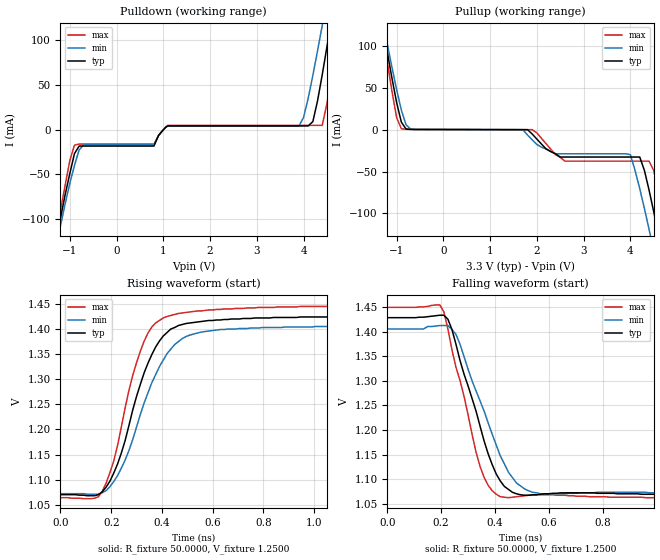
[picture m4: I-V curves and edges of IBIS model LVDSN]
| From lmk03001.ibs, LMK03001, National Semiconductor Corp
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|   Model LVDSN
[Model]  LVDSN
Model_type Output
Polarity   Inverting
Vmeas =  1.2780V
Rref =   50.0000
Vref =   1.2500V
C_comp   1.6000pF   1.6000pF   1.6000pF
[Temperature Range]   25.0000   85.0000   -40.0000
[Voltage Range]   3.3000V   3.1500V   3.4500V
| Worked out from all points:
|   slope of the pullup table from 0 to 0.495 V, typ, clamps not added: 9.98 kohm
|   rising waveform, R_fixture 50.0000, V_fixture 1.2500: 20-80 % time 134ps typ, 152ps min, 115ps max; typ from 1.07 V to 1.43 V
|   falling waveform, R_fixture 50.0000, V_fixture 1.2500: 20-80 % time 119ps typ, 137ps min, 101ps max; typ from 1.43 V to 1.07 V
[Pulldown]
|Voltage   I(typ)   I(min)   I(max)
-3.45V    -669.4mA   -638.7mA   -724mA
-1.3V     -126.3mA   -133.2mA   -120mA
-900mV    -26.71mA   -39.95mA   -17.23mA
-700mV    -18.3mA    -16.89mA   -16.07mA
800mV     -18.3mA    -16.89mA   -16.07mA
1.1V      4.237mA    3.877mA    4.82mA
3.9V      4.237mA    3.877mA    4.82mA
4.2V      9.056mA    60.8mA     4.82mA
4.4V      61.28mA    116.4mA    4.82mA
4.6V      124.2mA    174mA      63.07mA
4.8V      189.4mA    232.6mA    137mA
6.9V      832.6mA    800.9mA    875.6mA
[Pullup]
|Voltage   I(typ)   I(min)   I(max)
-3.45V    832.6mA    755.7mA    934.3mA
-1.3V     124.2mA    130.7mA    118.2mA
-900mV    9.056mA    23.5mA     1.096mA
-700mV    356.2uA    687.6uA    401.7uA
1.9V      -5.159mA   -12.12mA   33.99uA
2.6V      -32.65mA   -28.75mA   -37.57mA
4V        -32.65mA   -29.82mA   -37.57mA
4.2V      -32.65mA   -70.34mA   -37.57mA
4.4V      -72.21mA   -119.1mA   -37.57mA
4.6V      -125.3mA   -170.8mA   -75.8mA
4.8V      -181.4mA   -223.8mA   -134.7mA
6.9V      -666.4mA   -669.2mA   -681mA
[Ramp]
| variable   typ   min   max
dV/dt_r  0.2150/0.1345n   0.2004/0.1510n   0.2300/0.1137n
dV/dt_f  0.2172/0.1181n   0.2037/0.1385n   0.2318/0.1004n
R_load = 50.00
[Rising Waveform]
R_fixture= 50.0000
V_fixture= 1.2500
V_fixture_min= 1.2500
V_fixture_max= 1.2500
|time   V(typ)   V(min)   V(max)
0s        1.07V      1.072V     1.064V
165ps     1.076V     1.074V     1.077V
225ps     1.131V     1.108V     1.168V
270ps     1.208V     1.158V     1.278V
315ps     1.29V      1.23V      1.356V
360ps     1.349V     1.293V     1.404V
405ps     1.386V     1.338V     1.422V
480ps     1.409V     1.381V     1.432V
630ps     1.418V     1.399V     1.439V
1.485ns   1.426V     1.406V     1.448V
[Falling Waveform]
R_fixture= 50.0000
V_fixture= 1.2500
V_fixture_min= 1.2500
V_fixture_max= 1.2500
|time   V(typ)   V(min)   V(max)
0s        1.429V     1.406V     1.45V
195ps     1.434V     1.413V     1.455V
225ps     1.426V     1.413V     1.406V
255ps     1.375V     1.395V     1.328V
345ps     1.207V     1.259V     1.125V
375ps     1.151V     1.214V     1.087V
420ps     1.096V     1.147V     1.064V
480ps     1.07V      1.092V     1.064V
570ps     1.069V     1.07V      1.068V
1.485ns   1.069V     1.071V     1.06V
